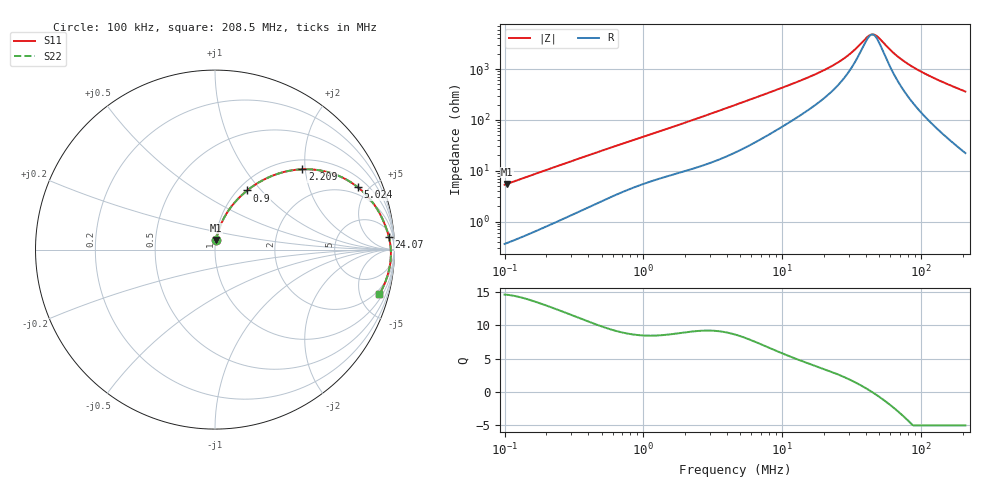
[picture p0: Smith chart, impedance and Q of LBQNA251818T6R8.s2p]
! LBQNA251818T6R8  S-PARAMETER MODEL  ( General Type )
! Model Generated by TAIYO YUDEN Corporation (http://www.ty-top.com)
! Version 1.0
! TAIYO YUDEN Control No. 191025NI43SB-FBB
! Copyright(c) 2019 TAIYO YUDEN CO.,LTD. All Rights Reserved.
! Product Description (link to TY-COMPAS)
! https://ds.yuden.co.jp/TYCOMPAS/or/detail?pn=LBQNA251818T6R8M&u=M
! Products Name : Inductors
! Characteristics :
!  Inductance : 6.8 uH , SRF(min) : 38 MHz , DC Resistance(max) : 0.195 Ohm
!  Rated Current : Saturation :270 mA , Temp Rise : 750 mA (20 degC)
!  Case Size : 2.5 x 1.8 / 0.098 x 0.071 [mm/inch] , Thickness : 1.8 / 0.071 [mm/inch]
!  (Conditions: Temperature = 25 degC , DC Bias Current/Voltage = 0A / 0V)
! External Node Assignments :
!  1  o---GGG---o  2
! GND o---------o GND
! Frequency Range : 0.1MHz  -  208.503118MHz  [ 402 STEP ]
# MHz S RI R 50
! Freq[MHz].  S11 Real  S11 Imag  S21 Real  S21 Imag  S12 Real  S12 Imag  S22 Real  S22 Imag
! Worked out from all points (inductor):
!   401 points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, 100 kHz to 208.5 MHz, reference 50 ohm
!   read as one part in series: L = 8.35 uH near 103.9 kHz
!   highest Q = 14.5 at 103.9 kHz (marker M1), where L = 8.4 uH
!   self-resonance near 44.32 MHz
!   S11 on the Smith chart (normalised r, x): 100 kHz: 1.01, +0.11; 900 kHz: 1.10, +0.84; 2.209 MHz: 1.21, +1.93; 5.024 MHz: 1.51, +4.28; 24.07 MHz: 9, +24; 208.5 MHz: 1.44, -7.22
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0.1  0.00637 0.0523  0.9936 -0.0523  0.9936 -0.0523  0.00637 0.0523
0.103895  0.00672 0.0542  0.9933 -0.0542  0.9933 -0.0542  0.00672 0.0542
0.359709  0.0464 0.1695  0.9536 -0.1695  0.9536 -0.1695  0.0464 0.1695
0.579957  0.097 0.2474  0.903 -0.2474  0.903 -0.2474  0.097 0.2474
0.900005  0.1795 0.3295  0.8205 -0.3295  0.8205 -0.3295  0.1795 0.3295
1.293906  0.281 0.3942  0.719 -0.3942  0.719 -0.3942  0.281 0.3942
2.209228  0.4867 0.4474  0.5133 -0.4474  0.5133 -0.4474  0.4867 0.4474
3.116023  0.632 0.4308  0.368 -0.4308  0.368 -0.4308  0.632 0.4308
4.654297  0.7742 0.3636  0.2258 -0.3636  0.2258 -0.3636  0.7742 0.3636
5.023949  0.7958 0.3474  0.2042 -0.3474  0.2042 -0.3474  0.7958 0.3474
8.415604  0.8972 0.2357  0.1028 -0.2357  0.1028 -0.2357  0.8972 0.2357
16.42508  0.9534 0.1209  0.0466 -0.1209  0.0466 -0.1209  0.9534 0.1209
24.06929  0.9685 0.0709  0.0315 -0.0709  0.0315 -0.0709  0.9685 0.0709
30.27169  0.9744 0.0437  0.0256 -0.0437  0.0256 -0.0437  0.9744 0.0437
40.31841  0.9788 0.0109  0.0212 -0.0109  0.0212 -0.0109  0.9788 0.0109
43.52056  0.9794 0.00209  0.0206 -0.00209  0.0206 -0.00209  0.9794 0.00209
47.88322  0.98 -0.00896  0.02 0.00896  0.02 0.00896  0.98 -0.00896
59.08252  0.98 -0.034  0.02 0.034  0.02 0.034  0.98 -0.034
72.90118  0.9782 -0.0607  0.0218 0.0607  0.0218 0.0607  0.9782 -0.0607
95.25845  0.9726 -0.0984  0.0274 0.0984  0.0274 0.0984  0.9726 -0.0984
136.9498  0.9564 -0.1596  0.0436 0.1596  0.0436 0.1596  0.9564 -0.1596
208.5031  0.9158 -0.2486  0.0842 0.2486  0.0842 0.2486  0.9158 -0.2486
